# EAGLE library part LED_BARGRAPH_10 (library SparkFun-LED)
Young Sun LED Tech - YSLB-10251G5-10 10-Segment LED Bar Graph Features: Red Vf = 2.1V, Ifmax = 20mA Yellow Vf = 2.1V, Ifmax = 20mA Blue Vf = 3.4V, Ifmax = 20mA Green Vf = 3.4V, Ifmax = 20mA SparkFun Products: Red Yellow Green Blue
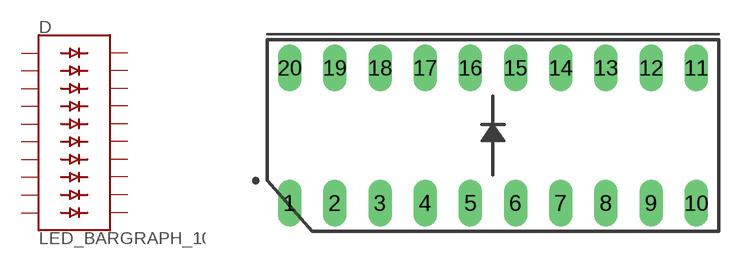
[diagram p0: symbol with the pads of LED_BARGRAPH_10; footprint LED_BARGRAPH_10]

Designator prefix D

## LED_BARGRAPH_10RED (PROD_ID: DIO-10615; VALUE: RED)  [LED_BARGRAPH_10]
1  A  pas
2  A1  pas
3  A2  pas
4  A3  pas
5  A4  pas
6  A5  pas
7  A6  pas
8  A7  pas
9  A8  pas
10  A9  pas
11  C9  pas
12  C8  pas
13  C7  pas
14  C6  pas
15  C5  pas
16  C4  pas
17  C3  pas
18  C2  pas
19  C1  pas
20  C  pas

## LED_BARGRAPH_10YELLOW (PROD_ID: DIO-10614; VALUE: YELLOW)  [LED_BARGRAPH_10]
Pads as for LED_BARGRAPH_10

## LED_BARGRAPH_10BLUE (PROD_ID: DIO-10613; VALUE: BLUE)  [LED_BARGRAPH_10]
Pads as for LED_BARGRAPH_10

## LED_BARGRAPH_10GREEN (PROD_ID: DIO-10612; VALUE: GREEN)  [LED_BARGRAPH_10]
Pads as for LED_BARGRAPH_10

## Footprint LED_BARGRAPH_10 (pad centres in mm)
10 Segment LED Bar Graph Specifications: Pin count: 20 Pin pitch: 1.74mm Area:10mm x 25.5mm Datasheet referenced for footprint: YSLB-102510B5
drill 0.813 long: 1 -11.43,-3.81; 2 -8.89,-3.81; 3 -6.35,-3.81; 4 -3.81,-3.81; 5 -1.27,-3.81; 6 1.27,-3.81; 7 3.81,-3.81; 8 6.35,-3.81; 9 8.89,-3.81; 10 11.43,-3.81; 11 11.43,3.81; 12 8.89,3.81; 13 6.35,3.81; 14 3.81,3.81; 15 1.27,3.81; 16 -1.27,3.81; 17 -3.81,3.81; 18 -6.35,3.81; 19 -8.89,3.81; 20 -11.43,3.81

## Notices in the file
Licensing: Creative Commons ShareAlike 4.0 International - https://creativecommons.org/licenses/by-sa/4.0
